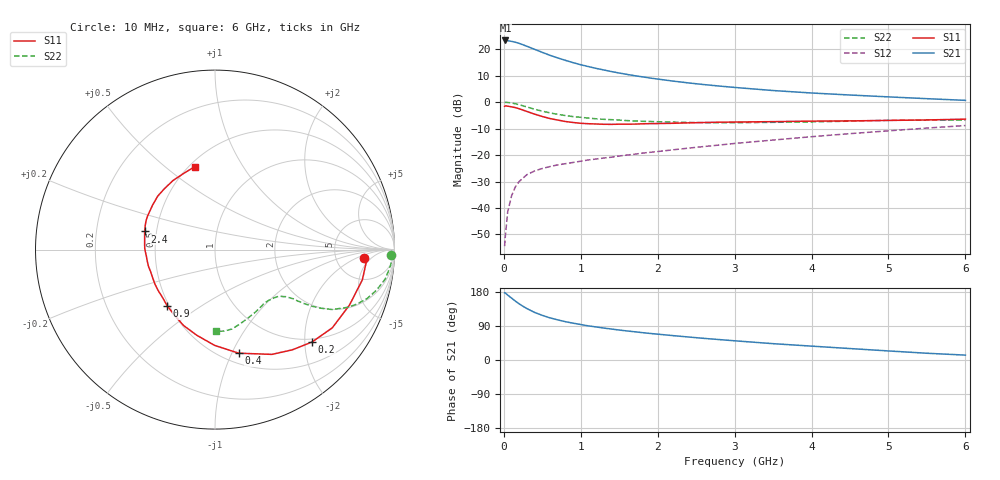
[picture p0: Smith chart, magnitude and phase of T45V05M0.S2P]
! Infineon Technologies  Discrete & RF Semiconductors
! BFR182T
! Si NPN RF Bipolar Junction Transistor in SC75
! VCE = 5 V  IC = 5 mA
! Common Emitter S-Parameters:  October  1999
# GHz  S  MA  R  50
!  f  S11  S21  S12  S22
! GHz  MAG  ANG  MAG  ANG  MAG  ANG  MAG  ANG
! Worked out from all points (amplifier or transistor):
!   36 points, 10 MHz to 6 GHz, reference 50 ohm
!   highest |S21| = 23.3 dB at 20 MHz (marker M1)
!   |S21| within 3 dB of that: start of sweep to 369.5 MHz
!   unconditionally stable (mu >= 1): 1.443 GHz to 4.053 GHz
!   at 250 MHz: K = 0.28, MSG = 25.2 dB, |S12| = -28.7 dB
!   at 1.4 GHz: K = 0.99, MSG = 16.2 dB, |S12| = -20.8 dB
!   at 6 GHz: K = 0.84, MSG = 4.8 dB, |S12| = -8.9 dB
!   lowest NFmin = 1.20 dB at 450 MHz
!   S11 on the Smith chart (normalised r, x): 10 MHz: 10, -3; 200 MHz: 0.93, -2.16; 400 MHz: 0.60, -1.06; 900 MHz: 0.49, -0.37; 2.4 GHz: 0.43, +0.10; 6 GHz: 0.53, +0.64
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0.01  0.8314 -3.4  14.47 177.3  0.0019 86.0  0.9825 -1.8
0.02  0.8486 -3.4  14.57 176.7  0.003 88.2  0.9889 -2.0
0.05  0.8381 -11.6  14.41 171.3  0.0084 89.7  0.9825 -5.1
0.1  0.8106 -22.4  14.01 163.4  0.0169 80.0  0.9628 -9.8
0.15  0.7855 -33.7  13.49 155.3  0.0251 72.9  0.9278 -14.1
0.2  0.7465 -43.6  12.83 148.1  0.0317 70.3  0.8906 -17.8
0.25  0.7051 -52.4  12.05 141.6  0.0368 65.1  0.8484 -20.9
0.3  0.6643 -61.5  11.31 135.7  0.0426 62.5  0.8089 -23.4
0.4  0.5921 -77.1  9.907 125.5  0.05 57.5  0.733 -27.1
0.5  0.5338 -90.2  8.675 117.8  0.0557 55.2  0.6734 -29.0
0.6  0.488 -102.0  7.638 111.2  0.0606 53.4  0.6249 -30.3
0.7  0.4577 -112.5  6.822 105.9  0.0651 52.4  0.5862 -31.1
0.8  0.4296 -121.7  6.14 101.1  0.0686 52.4  0.5561 -31.6
0.9  0.4116 -130.2  5.551 97.2  0.0724 53.0  0.5316 -32.0
1.1  0.39 -144.7  4.676 90.0  0.0808 53.6  0.498 -32.8
1.6  0.383 -171.0  3.331 76.7  0.0998 56.5  0.4471 -35.5
2.2  0.3976 170.2  2.489 64.3  0.1255 59.5  0.4191 -41.0
2.4  0.4047 165.5  2.299 60.7  0.1349 60.4  0.4117 -43.3
3.5  0.4269 144.6  1.651 43.1  0.1918 61.1  0.4144 -56.9
4.5  0.4411 129.7  1.359 30.2  0.2534 58.8  0.4359 -70.9
5.5  0.4594 112.1  1.159 17.8  0.3231 54.4  0.4568 -83.6
6  0.476 103.5  1.077 12.9  0.3604 51.2  0.4557 -89.0
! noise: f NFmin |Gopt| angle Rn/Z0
0.45  1.2  0.27  37  0.3
0.9  1.3  0.25  75  0.23
1.8  1.9  0.21  145  0.2
